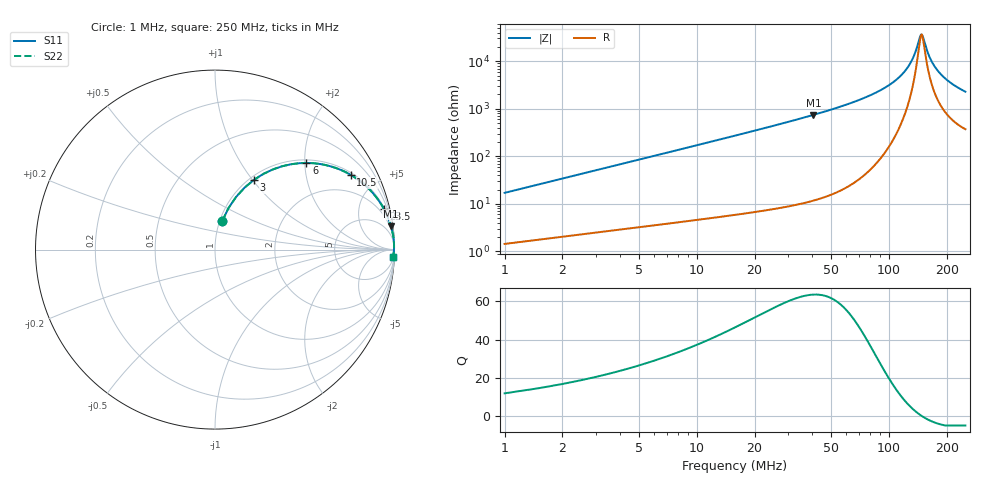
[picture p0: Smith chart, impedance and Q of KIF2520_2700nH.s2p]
!version-2
!date-12.2020
!Series
# MHz S RI R 50
!Freq ReS11 ImS11 ReS21 ImS21 ReS12 ImS12 ReS22 ImS22
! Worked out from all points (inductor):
!   499 points, 1 MHz to 250 MHz, reference 50 ohm
!   read as one part in series: L = 2.7 uH near 2 MHz
!   highest Q = 63.5 at 40.5 MHz (marker M1), where L = 2.92 uH
!   self-resonance near 147.5 MHz
!   S11 on the Smith chart (normalised r, x): 1 MHz: 1.03, +0.34; 3 MHz: 1.05, +1.02; 6 MHz: 1.07, +2.04; 10.5 MHz: 1.09, +3.58; 23.5 MHz: 1.15, +8.18; 250 MHz: 8, -45
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1  0.041 0.1604  0.959 -0.1604  0.959 -0.1604  0.041 0.1604
3  0.2174 0.3888  0.7826 -0.3888  0.7826 -0.3888  0.2174 0.3888
4.5  0.3739 0.4643  0.6261 -0.4643  0.6261 -0.4643  0.3739 0.4643
6  0.5096 0.4829  0.4904 -0.4829  0.4904 -0.4829  0.5096 0.4829
8  0.6455 0.4636  0.3545 -0.4636  0.3545 -0.4636  0.6455 0.4636
10.5  0.7566 0.4162  0.2434 -0.4162  0.2434 -0.4162  0.7566 0.4162
15.5  0.8708 0.3247  0.1292 -0.3247  0.1292 -0.3247  0.8708 0.3247
23.5  0.9399 0.2287  0.0601 -0.2287  0.0601 -0.2287  0.9399 0.2287
40.5  0.9802 0.1316  0.0198 -0.1316  0.0198 -0.1316  0.9802 0.1316
42.5  0.9822 0.1247  0.0178 -0.1247  0.0178 -0.1247  0.9822 0.1247
84  0.9963 0.0473  0.00368 -0.0473  0.00368 -0.0473  0.9963 0.0473
109  0.9976 0.0246  0.00238 -0.0246  0.00238 -0.0246  0.9976 0.0246
125.5  0.9977 0.0131  0.0023 -0.0131  0.0023 -0.0131  0.9977 0.0131
135  0.9976 0.00727  0.00242 -0.00727  0.00242 -0.00727  0.9976 0.00727
145  0.9973 0.00161  0.00265 -0.00161  0.00265 -0.00161  0.9973 0.00161
147.5  0.9973 0.000261  0.00272 -0.000261  0.00272 -0.000261  0.9973 0.000261
150  0.9972 -0.00107  0.0028 0.00107  0.0028 0.00107  0.9972 -0.00107
160  0.9968 -0.00616  0.00316 0.00616  0.00316 0.00616  0.9968 -0.00616
167  0.9965 -0.00954  0.00345 0.00954  0.00345 0.00954  0.9965 -0.00954
184  0.9957 -0.0172  0.00429 0.0172  0.00429 0.0172  0.9957 -0.0172
208.5  0.9942 -0.0273  0.00577 0.0273  0.00577 0.0273  0.9942 -0.0273
250  0.9911 -0.0425  0.0089 0.0425  0.0089 0.0425  0.9911 -0.0425
